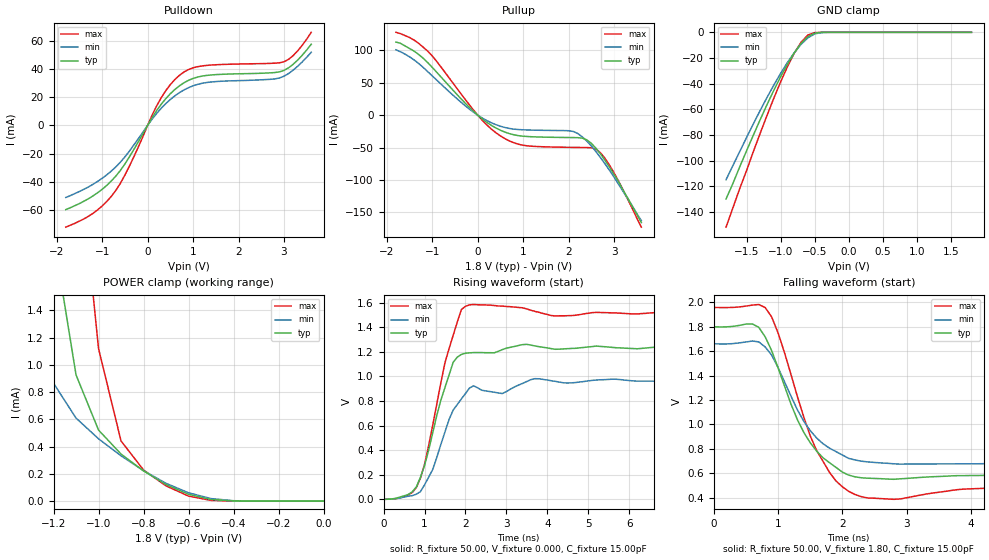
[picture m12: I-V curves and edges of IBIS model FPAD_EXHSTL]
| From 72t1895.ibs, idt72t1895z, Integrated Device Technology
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|   Model FPAD_EXHSTL
[Model]   FPAD_EXHSTL
Model_type   3-state
Polarity   Non-Inverting
Enable   Active-Low
Vmeas =  0.900V
C_comp   3.00pF   NA   NA
[Temperature Range]   25.00   85.00   -40.00
[Voltage Range]   1.80V   1.60V   2.00V
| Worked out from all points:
|   slope of the pulldown table from 0 to 0.27 V, typ, clamps not added: 19.7 ohm
|   slope of the pullup table from 0 to 0.27 V, typ, clamps not added: 18.8 ohm
|   GND clamp passes 1 mA (typ) near -0.51 V on its own axis
|   POWER clamp passes 1 mA (typ) near -1.11 V on its own axis
|   rising waveform, R_fixture 50.00, V_fixture 0.000, C_fixture 15.00pF: 20-80 % time 605ps typ, 680ps min, 575ps max; typ from 0 V to 1.23 V
|   falling waveform, R_fixture 50.00, V_fixture 1.80, C_fixture 15.00pF: 20-80 % time 604ps typ, 627ps min, 570ps max; typ from 1.8 V to 0.58 V
[Pulldown]
| voltage   I(typ)   I(min)   I(max)
-1.8V     -59.8mA    -51.2mA    -72.3mA
-1.2V     -50.07mA   -41.81mA   -62.46mA
-700mV    -36.05mA   -29.51mA   -46.23mA
-400mV    -22.33mA   -18.22mA   -28.88mA
200mV     10.57mA    8.525mA    13.92mA
400mV     19.01mA    15.49mA    24.67mA
700mV     28.12mA    23.26mA    35.58mA
900mV     32.02mA    26.81mA    39.69mA
1.2V      35.04mA    29.92mA    42.26mA
3V        39.06mA    34.94mA    45.2mA
3.3V      46.36mA    41.95mA    52.89mA
3.6V      57.64mA    51.96mA    66.13mA
[Pullup]
| voltage   I(typ)   I(min)   I(max)
-1.8V     113mA      101mA      128mA
-1.4V     98.92mA    85.36mA    116mA
-1.1V     81.21mA    67.28mA    98.93mA
-100mV    6.412mA    4.931mA    8.552mA
500mV     -23.29mA   -17.11mA   -32.09mA
1V        -32.5mA    -22.62mA   -46.53mA
2.2V      -34.74mA   -28.29mA   -49.87mA
2.4V      -38.17mA   -40.02mA   -50.05mA
2.6V      -51.02mA   -56.23mA   -52.33mA
2.8V      -69.73mA   -75.15mA   -66.69mA
3.1V      -103mA     -107mA     -102mA
3.6V      -166mA     -163mA     -173mA
[GND_clamp]
| voltage   I(typ)   I(min)   I(max)
-1.8V     -130mA     -115mA     -152mA
-1.6V     -105mA     -93.09mA   -122mA
-1.3V     -68.22mA   -61mA      -78.85mA
-1.1V     -45.3mA    -41.22mA   -51.5mA
-1V       -34.68mA   -32.07mA   -38.72mA
-900mV    -24.85mA   -23.59mA   -26.87mA
-800mV    -16.08mA   -15.96mA   -16.35mA
-700mV    -8.721mA   -9.411mA   -7.76mA
-600mV    -3.357mA   -4.326mA   -2.135mA
-500mV    -667uA     -1.241mA   -218uA
-400mV    -58.99uA   -179uA     -9.374uA
1.8V      18.04nA    37.81nA    18nA
[POWER_clamp]
| voltage   I(typ)   I(min)   I(max)
-1.8V     20.11mA    12.65mA    31.29mA
-1.3V     3.744mA    1.476mA    8.598mA
-1.2V     1.95mA     866uA      5.327mA
-1.1V     927uA      610uA      2.766mA
-1V       522uA      458uA      1.121mA
-900mV    346uA      333uA      442uA
-800mV    222uA      224uA      229uA
-700mV    122uA      131uA      112uA
-600mV    50.35uA    61.27uA    37.19uA
-500mV    11.87uA    18.7uA     5.408uA
-400mV    1.361uA    3.089uA    377nA
0V        18.04nA    17.69nA    20nA
[Ramp]
| variable   typ   min   max
dV/dt_r   0.75/0.33n   0.58/0.34n   0.92/0.33n
dV/dt_f   0.74/0.25n   0.61/0.25n   0.89/0.28n
R_load = 50.00
[Rising Waveform]
R_fixture = 50.00
V_fixture = 0.000
C_fixture = 15.00pF
R_dut = 0.75
L_dut = 8.10nH
C_dut = 0.53pF
| time   V(typ)   V(min)   V(max)
0s        0V         0V         0V
600ps     39.4mV     24.93mV    36.09mV
900ps     180mV      62.74mV    173mV
1.2ns     542mV      243mV      604mV
1.5ns     910mV      549mV      1.112V
1.7ns     1.114V     726mV      1.334V
2ns       1.188V     860mV      1.569V
2.9ns     1.217V     860mV      1.571V
3.7ns     1.247V     981mV      1.528V
9.9ns     1.232V     964mV      1.513V
[Falling Waveform]
R_fixture = 50.00
V_fixture = 1.80
C_fixture = 15.00pF
R_dut = 0.75
L_dut = 8.10nH
C_dut = 0.53pF
| time   V(typ)   V(min)   V(max)
0s        1.8V       1.66V      1.958V
600ps     1.823V     1.683V     1.977V
800ps     1.717V     1.634V     1.957V
1ns       1.464V     1.466V     1.75V
1.3ns     1.04V      1.121V     1.23V
1.6ns     782mV      889mV      787mV
1.9ns     649mV      778mV      538mV
2.3ns     563mV      699mV      408mV
4.3ns     583mV      679mV      479mV
9.9ns     580mV      679mV      465mV
